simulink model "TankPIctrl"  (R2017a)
settings: Solver=ode15s  StartTime=0.0  StopTime=100  RelTol=1e-3
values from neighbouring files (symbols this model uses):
  d1amplitude = 0.05    [ExamplePIbased.m]    (also in levelcontrol_init3.m; levelcontrol_init4.m; levelcontrol_init5.m; levelcontrol_init6.m)
  d1bias = 0    [ExamplePIbased.m]    (also in levelcontrol_init3.m; levelcontrol_init4.m; levelcontrol_init5.m; levelcontrol_init6.m)
  d1freq = 1    [ExamplePIbased.m]    (also in levelcontrol_init3.m; levelcontrol_init4.m; levelcontrol_init5.m; levelcontrol_init6.m)
  d1phase = 0    [ExamplePIbased.m]    (also in levelcontrol_init3.m; levelcontrol_init4.m; levelcontrol_init5.m; levelcontrol_init6.m)
  d2 = 0.4    [ExamplePIbased.m]    (also in levelcontrol_init3.m = 0.2; levelcontrol_init4.m = 0.2; levelcontrol_init5.m; levelcontrol_init6.m = 0.2)
  d3 = -0.8    [ExamplePIbased.m]    (also in levelcontrol_init3.m = 0.2; levelcontrol_init4.m = 0.2; levelcontrol_init5.m; levelcontrol_init6.m = 0.2)
  d4 = 0.05    [ExamplePIbased.m]    (also in levelcontrol_init3.m = 0.1; levelcontrol_init4.m; levelcontrol_init5.m; levelcontrol_init6.m)
  d5 = -0.9    [ExamplePIbased.m]    (also in levelcontrol_init3.m; levelcontrol_init4.m; levelcontrol_init5.m; levelcontrol_init6.m)
  h0 = 0.5    [ExamplePIbased.m]    (also in levelcontrol_init3.m; levelcontrol_init4.m; levelcontrol_init5.m; levelcontrol_init6.m)
  h_set = 0.5    [ExamplePIbased.m]    (also in levelcontrol_init3.m; levelcontrol_init4.m; levelcontrol_init5.m; levelcontrol_init6.m)
  Kc = (1/kprime)*(1/(tau_c+theta))    (= -0.333333333333)    [ExamplePIbased.m]    (also in levelcontrol_init3.m; levelcontrol_init4.m; levelcontrol_init5.m; levelcontrol_init6.m)
  noise_ON = 0    [ExamplePIbased.m]    (also in levelcontrol_init3.m = 1; levelcontrol_init4.m; levelcontrol_init5.m; levelcontrol_init6.m = 1)
  p = 1    [ExamplePIbased.m]    (also in levelcontrol_init3.m; levelcontrol_init4.m; levelcontrol_init5.m; levelcontrol_init6.m)
  qin0 = 0.5    [ExamplePIbased.m]    (also in levelcontrol_init3.m; levelcontrol_init4.m; levelcontrol_init5.m; levelcontrol_init6.m)
  qout0 = 0.5    [ExamplePIbased.m]    (also in levelcontrol_init3.m; levelcontrol_init4.m; levelcontrol_init5.m; levelcontrol_init6.m)
  sin_ON = 1    [ExamplePIbased.m]    (also in levelcontrol_init3.m; levelcontrol_init4.m = 0; levelcontrol_init5.m; levelcontrol_init6.m)
  tauI = 4*(tau_c+theta)    (= 12)    [ExamplePIbased.m]    (also in levelcontrol_init3.m; levelcontrol_init4.m; levelcontrol_init5.m; levelcontrol_init6.m)
  td2 = 30    [ExamplePIbased.m]    (also in levelcontrol_init3.m = 50; levelcontrol_init4.m = 50; levelcontrol_init5.m; levelcontrol_init6.m = 50)
  td3 = 200    [ExamplePIbased.m]    (also in levelcontrol_init3.m = 100; levelcontrol_init4.m = 100; levelcontrol_init5.m; levelcontrol_init6.m = 100)
  td4 = 350    [ExamplePIbased.m]    (also in levelcontrol_init3.m = 150; levelcontrol_init4.m = 150; levelcontrol_init5.m; levelcontrol_init6.m = 150)
  td5 = 300    [ExamplePIbased.m]    (also in levelcontrol_init3.m = 200; levelcontrol_init4.m = 205; levelcontrol_init5.m; levelcontrol_init6.m = 205)
  Umax = 1    [ExamplePIbased.m]    (also in levelcontrol_init3.m; levelcontrol_init4.m; levelcontrol_init5.m; levelcontrol_init6.m)
  Umaxsat = Umax-qout0    (= 0.5)    [ExamplePIbased.m]    (also in levelcontrol_init3.m; levelcontrol_init4.m; levelcontrol_init5.m; levelcontrol_init6.m)
  Umin = 0    [ExamplePIbased.m]    (also in levelcontrol_init3.m; levelcontrol_init4.m; levelcontrol_init5.m; levelcontrol_init6.m)
  Uminsat = Umin-qout0    (= -0.5)    [ExamplePIbased.m]    (also in levelcontrol_init3.m; levelcontrol_init4.m; levelcontrol_init5.m; levelcontrol_init6.m)
undefined symbols (not defined in the file or in its folder): SimpleTank_ODE
libraries: simulink x2

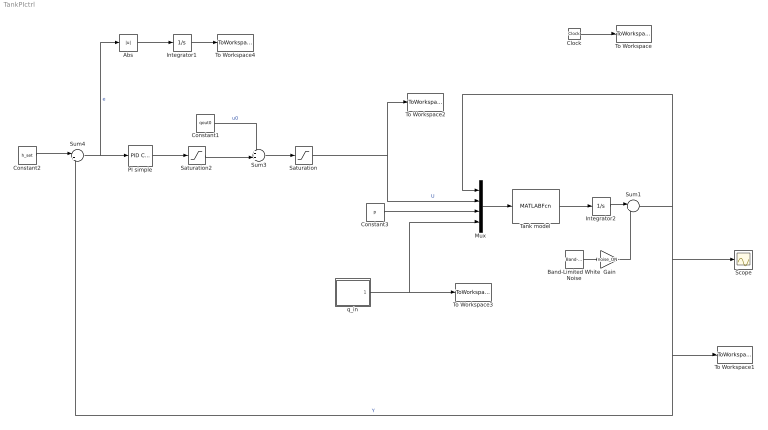
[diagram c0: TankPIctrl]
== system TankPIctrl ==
  Abs : Abs
  Band-Limited White Noise : simulink/Sources/Band-Limited White Noise  Cov=noise_power  Ts=0.1  seed=[23341]
  Clock : Clock
  Constant1 : Constant  Value=qout0
  Constant2 : Constant  Value=h_set
  Constant3 : Constant  Value=p
  Gain : Gain  Gain=noise_ON
  Integrator1 : Integrator
  Integrator2 : Integrator  InitialCondition=h0
  Mux : Mux
  PI simple : simulink/Continuous/PID Controller  Controller=PI  TimeDomain=Continuous-time  SampleTime=-1  IntegratorMethod=Forward Euler  FilterMethod=Forward Euler  Form=Parallel  UseFilter=on  ControllerParametersSource=internal  P=Kc  I=Kc/tauI  D=0  N=100  InitialConditionSource=internal  InitialConditionForIntegrator=0  InitialConditionForFilter=0  ExternalReset=none  LimitOutput=on  UpperSaturationLimit=Umaxsat  LowerSaturationLimit=Uminsat  LinearizeAsGain=on  AntiWindupMode=back-calculation  Kb=1  TrackingMode=off  Kt=1  PParamMin=[]  PParamMax=[]  IParamMin=[]  IParamMax=[]  DParamMin=[]  DParamMax=[]  NParamMin=[]  NParamMax=[]  KbParamMin=[]  KbParamMax=[]  KtParamMin=[]  KtParamMax=[]  POutMin=[]  POutMax=[]  IOutMin=[]  IOutMax=[]  DOutMin=[]  DOutMax=[]  NOutMin=[]  NOutMax=[]  KbOutMin=[]  KbOutMax=[]  KtOutMin=[]  KtOutMax=[]  IntegratorOutMin=[]  IntegratorOutMax=[]  FilterOutMin=[]  FilterOutMax=[]  SumOutMin=[]  SumOutMax=[]  SumI1OutMin=[]  SumI1OutMax=[]  SumI2OutMin=[]  SumI2OutMax=[]  SumI3OutMin=[]  SumI3OutMax=[]  SumDOutMin=[]  SumDOutMax=[]  SaturationOutMin=[]  SaturationOutMax=[]  IntegratorContinuousStateAttributes=''  IntegratorStateMustResolveToSignalObject=off  IntegratorRTWStateStorageClass=Auto  FilterContinuousStateAttributes=''  FilterStateMustResolveToSignalObject=off  FilterRTWStateStorageClass=Auto  DifferentiatorICPrevScaledInput=0  DifferentiatorOutMin=[]  DifferentiatorOutMax=[]  InitialConditionSetting=State (most efficient)
  Saturation : Saturate  UpperLimit=Umax  LowerLimit=Umin
  Saturation2 : Saturate  UpperLimit=Umaxsat  LowerLimit=Uminsat
  Scope : Scope
  Sum1 : Sum  Inputs=|++
  Sum3 : Sum  Inputs=++|
  Sum4 : Sum  Inputs=|+-
  Tank model : MATLABFcn  MATLABFcn=SimpleTank_ODE(u(1),u(2),u(3),u(4))  OutputDimensions=1
  To Workspace : ToWorkspace  VariableName=time  SampleTime=-1
  To Workspace1 : ToWorkspace  VariableName=h  SaveFormat=Structure With Time  SampleTime=-1
  To Workspace2 : ToWorkspace  VariableName=q_out  SaveFormat=Structure With Time  SampleTime=-1
  To Workspace3 : ToWorkspace  VariableName=q_in  SaveFormat=Structure With Time  SampleTime=-1
  To Workspace4 : ToWorkspace  VariableName=IAE_PI  SaveFormat=Structure With Time  SampleTime=-1
  q_in : Subsystem
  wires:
  Clock/1 -> To Workspace/1
  Sum1/1 -> Mux/1, Sum4/2, To Workspace1/1, Scope/1  "Y"
  Saturation/1 -> Mux/2, To Workspace2/1  "U"
  Sum3/1 -> Saturation/1
  Constant1/1 -> Sum3/1  "u0"
  Constant2/1 -> Sum4/1
  Tank model/1 -> Integrator2/1
  Mux/1 -> Tank model/1
  Constant3/1 -> Mux/3
  Sum4/1 -> Abs/1, PI simple/1  "e"
  Saturation2/1 -> Sum3/2
  PI simple/1 -> Saturation2/1
  q_in/1(q_in) -> To Workspace3/1, Mux/4
  Integrator1/1 -> To Workspace4/1
  Abs/1 -> Integrator1/1
  Integrator2/1 -> Sum1/1
  Band-Limited White Noise/1 -> Gain/1
  Gain/1 -> Sum1/2

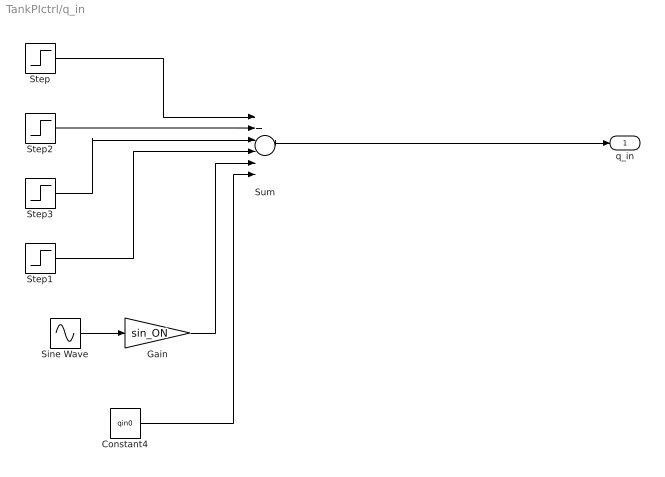
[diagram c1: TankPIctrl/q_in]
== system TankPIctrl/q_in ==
  Constant4 : Constant  Value=qin0
  Gain : Gain  Gain=sin_ON
  Sine Wave : Sin  Amplitude=d1amplitude  Bias=d1bias  Frequency=d1freq  Phase=d1phase  SampleTime=0
  Step : Step  Time=td2  After=d2  SampleTime=0
  Step1 : Step  Time=td5  After=d5  SampleTime=0
  Step2 : Step  Time=td3  After=d3  SampleTime=0
  Step3 : Step  Time=td4  After=d4  SampleTime=0
  Sum : Sum  Inputs=6
  q_in : Outport
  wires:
  Sum/1 -> q_in/1
  Step/1 -> Sum/1
  Step1/1 -> Sum/4
  Sine Wave/1 -> Gain/1
  Gain/1 -> Sum/5
  Step2/1 -> Sum/2
  Step3/1 -> Sum/3
  Constant4/1 -> Sum/6
